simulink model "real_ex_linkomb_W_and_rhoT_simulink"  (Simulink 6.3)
settings: Solver=ode45  StartTime=0.0  StopTime=simtid  RelTol=1e-3
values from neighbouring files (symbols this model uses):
  alpha = -0.9    [bounds.m]    (also in real_ex_linkomb_W_and_DP.m = 1; real_ex_linkomb_W_and_RHOT.m = -0.2; real_ex_without_noise_z_30.m = -6:0.01:4; toy_ex_nytt_system.m)
  K_indre = 10    [real_ex_linkomb_W_and_DP.m]    (also in real_ex_linkomb_W_and_RHOT.m = 5; toy_ex_nytt_system.m = 50; toy_ex_nytt_system_without_noise.m = 20; toy_ex_nytt_system_with_disturbance.m = 50)
  K_ytre = 0.01    [real_ex_linkomb_W_and_DP.m]    (also in real_ex_linkomb_W_and_RHOT.m; toy_ex_nytt_system.m = 0.1; toy_ex_nytt_system_without_noise.m = 0.1; toy_ex_nytt_system_with_disturbance.m = 0.1)
  Ti = 100    [real_ex_linkomb_W_and_DP.m]    (also in real_ex_linkomb_W_and_RHOT.m = 100000; toy_ex_nytt_system.m = 10; toy_ex_nytt_system_without_noise.m = 10; toy_ex_nytt_system_with_disturbance.m = 10)
undefined symbols (not defined in the file or in its folder): den_rhoT_tf, den_Wtf, num_rhoT_tf, num_Wtf

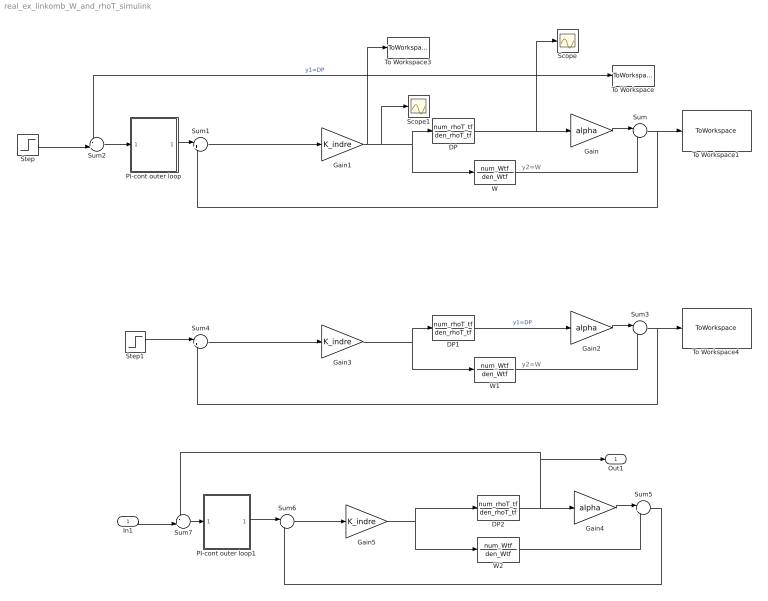
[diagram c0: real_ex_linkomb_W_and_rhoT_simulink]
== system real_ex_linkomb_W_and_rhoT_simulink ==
  note: y2=W
  note: y2=W
  In1 : Inport
  DP : TransferFcn  Numerator=num_rhoT_tf  Denominator=den_rhoT_tf
  DP1 : TransferFcn  Numerator=num_rhoT_tf  Denominator=den_rhoT_tf
  DP2 : TransferFcn  Numerator=num_rhoT_tf  Denominator=den_rhoT_tf
  Gain : Gain  Gain=alpha
  Gain1 : Gain  Gain=K_indre
  Gain2 : Gain  Gain=alpha
  Gain3 : Gain  Gain=K_indre
  Gain4 : Gain  Gain=alpha
  Gain5 : Gain  Gain=K_indre
  PI-cont outer loop : Subsystem
  PI-cont outer loop1 : Subsystem
  Scope : Scope
  Scope1 : Scope
  Step : Step  Time=0  SampleTime=0
  Step1 : Step  Time=1000  SampleTime=0
  Sum : Sum  Inputs=|++
  Sum1 : Sum  Inputs=|+-
  Sum2 : Sum  Inputs=-+|
  Sum3 : Sum  Inputs=|++
  Sum4 : Sum  Inputs=|+-
  Sum5 : Sum  Inputs=|++
  Sum6 : Sum  Inputs=|+-
  Sum7 : Sum  Inputs=-+|
  To Workspace : ToWorkspace  VariableName=simout_rhoT_tf  SampleTime=-1  SaveFormat=Structure With Time
  To Workspace1 : ToWorkspace  VariableName=simout_linkomb  SampleTime=-1  SaveFormat=Structure With Time
  To Workspace3 : ToWorkspace  VariableName=paadrag  SampleTime=-1  SaveFormat=Structure With Time
  To Workspace4 : ToWorkspace  VariableName=simout_linkomb_linkombonly  SampleTime=-1  SaveFormat=Structure With Time
  W : TransferFcn  Numerator=num_Wtf  Denominator=den_Wtf
  W1 : TransferFcn  Numerator=num_Wtf  Denominator=den_Wtf
  W2 : TransferFcn  Numerator=num_Wtf  Denominator=den_Wtf
  Out1 : Outport
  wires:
  DP/1 -> Gain/1, Sum2/1, To Workspace/1, Scope/1  "y1=DP"
  W/1 -> Sum/2
  Gain/1 -> Sum/1
  Gain1/1 -> DP/1, W/1, Scope1/1, To Workspace3/1
  Sum/1 -> Sum1/2, To Workspace1/1
  Step/1 -> Sum2/2
  Sum2/1 -> PI-cont outer loop/1(In1)
  PI-cont outer loop/1(Out1) -> Sum1/1
  Sum1/1 -> Gain1/1
  DP2/1 -> Gain4/1, Sum7/1, Out1/1
  W2/1 -> Sum5/2
  Gain4/1 -> Sum5/1
  Gain5/1 -> W2/1, DP2/1
  Sum5/1 -> Sum6/2
  Sum6/1 -> Gain5/1
  In1/1 -> Sum7/2
  Sum7/1 -> PI-cont outer loop1/1(In1)
  PI-cont outer loop1/1(Out1) -> Sum6/1
  DP1/1 -> Gain2/1  "y1=DP"
  W1/1 -> Sum3/2
  Gain2/1 -> Sum3/1
  Gain3/1 -> W1/1, DP1/1
  Sum3/1 -> To Workspace4/1, Sum4/2
  Step1/1 -> Sum4/1
  Sum4/1 -> Gain3/1

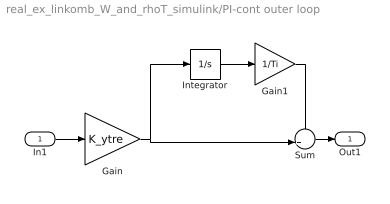
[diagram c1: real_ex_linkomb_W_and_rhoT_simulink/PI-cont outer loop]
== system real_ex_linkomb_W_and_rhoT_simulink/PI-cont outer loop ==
  In1 : Inport
  Gain : Gain  Gain=K_ytre
  Gain1 : Gain  Gain=1/Ti
  Integrator : Integrator
  Sum : Sum  Inputs=++|
  Out1 : Outport
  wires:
  Gain/1 -> Integrator/1, Sum/2
  In1/1 -> Gain/1
  Integrator/1 -> Gain1/1
  Gain1/1 -> Sum/1
  Sum/1 -> Out1/1

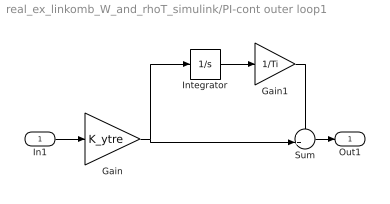
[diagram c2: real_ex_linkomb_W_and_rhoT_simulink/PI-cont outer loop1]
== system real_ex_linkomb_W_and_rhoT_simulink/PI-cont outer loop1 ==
  In1 : Inport
  Gain : Gain  Gain=K_ytre
  Gain1 : Gain  Gain=1/Ti
  Integrator : Integrator
  Sum : Sum  Inputs=++|
  Out1 : Outport
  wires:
  Sum/1 -> Out1/1
  Gain1/1 -> Sum/1
  Integrator/1 -> Gain1/1
  In1/1 -> Gain/1
  Gain/1 -> Sum/2, Integrator/1
